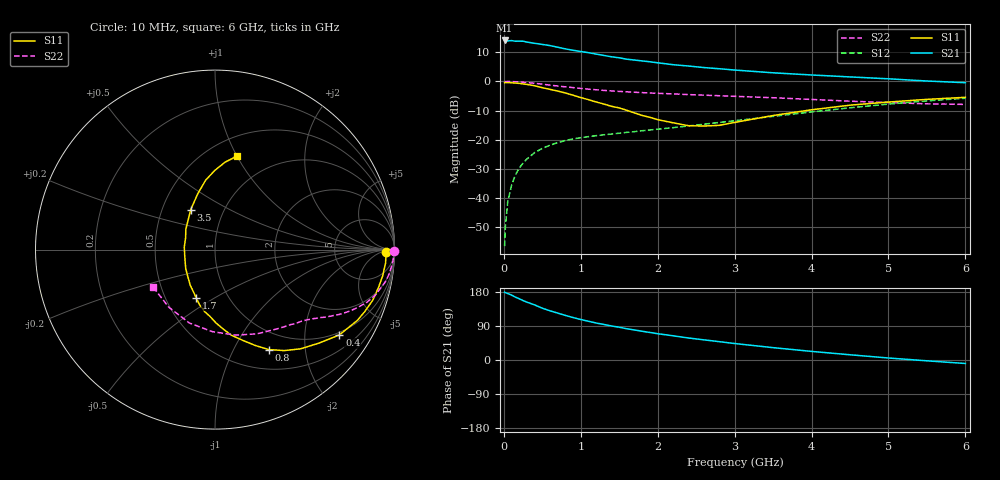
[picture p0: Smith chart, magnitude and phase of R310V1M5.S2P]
! SIEMENS Small Signal Semiconductors
! BFR181
! Si NPN RF Bipolar Junction Transistor in SOT23
! VCE = 10 V  IC = 1.5 mA
! Common Emitter S-Parameters:  May  1996
# GHz  S  MA  R  50
!  f  S11  S21  S12  S22
! GHz  MAG  ANG  MAG  ANG  MAG  ANG  MAG  ANG
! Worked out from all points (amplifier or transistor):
!   36 points, 10 MHz to 6 GHz, reference 50 ohm
!   highest |S21| = 14.0 dB at 10 MHz (marker M1)
!   |S21| within 3 dB of that: start of sweep to 824.1 MHz
!   unconditionally stable (mu >= 1): 1.875 GHz to 3.617 GHz
!   at 250 MHz: K = 0.19, MSG = 20.9 dB, |S12| = -28.0 dB
!   at 1.4 GHz: K = 0.86, MSG = 13.2 dB, |S12| = -18.1 dB
!   at 6 GHz: K = 0.86, MSG = 2.7 dB, |S12| = -5.8 dB
!   S11 on the Smith chart (normalised r, x): 10 MHz: 38, -12; 400 MHz: 0.92, -2.97; 800 MHz: 0.75, -1.39; 1.7 GHz: 0.71, -0.41; 3.5 GHz: 0.70, +0.33; 6 GHz: 0.69, +0.99
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0.01  0.9533 -0.9  5.021 178.9  0.0015 90.1  0.9976 -0.5
0.02  0.9537 -1.8  4.935 177.7  0.0032 91.8  0.9864 -0.9
0.05  0.9531 -4.6  4.933 175.5  0.0085 85.1  0.9964 -2.2
0.1  0.9455 -8.9  4.994 171.2  0.0165 84.4  0.9916 -4.3
0.15  0.935 -13.1  4.871 165.9  0.0248 80.9  0.9843 -6.6
0.25  0.9025 -22.6  4.87 156.9  0.0399 75.7  0.9663 -10.7
0.4  0.8406 -34.4  4.49 145.4  0.0601 69.2  0.9282 -15.9
0.5  0.7789 -42.0  4.294 136.7  0.071 65.2  0.8961 -19.1
0.6  0.7295 -49.3  4.099 129.9  0.0806 61.6  0.8614 -21.8
0.8  0.6327 -61.7  3.602 117.7  0.0969 56.4  0.805 -25.9
0.9  0.5788 -67.3  3.409 112.0  0.1031 54.5  0.7817 -27.5
1.1  0.4855 -79.2  3.101 102.2  0.1129 52.0  0.7359 -30.4
1.2  0.4434 -84.3  2.935 97.6  0.1174 51.1  0.7172 -31.7
1.4  0.3732 -94.3  2.637 89.8  0.1251 50.5  0.6855 -33.9
1.7  0.2877 -111.5  2.316 79.2  0.1376 50.2  0.6505 -36.8
2  0.2205 -132.1  2.08 69.4  0.1514 50.9  0.6239 -39.9
2.2  0.195 -146.7  1.929 63.9  0.161 51.4  0.6097 -42.4
2.8  0.1763 158.4  1.645 48.4  0.1976 53.0  0.5673 -50.4
3.5  0.2601 121.3  1.401 32.6  0.2511 51.9  0.5241 -63.6
4.5  0.3908 97.6  1.191 13.8  0.3525 45.6  0.4574 -91.8
5.5  0.4913 83.3  1.014 -2.2  0.4625 34.0  0.4116 -128.7
6  0.5331 77.0  0.948 -9.2  0.5138 26.8  0.4029 -148.8
